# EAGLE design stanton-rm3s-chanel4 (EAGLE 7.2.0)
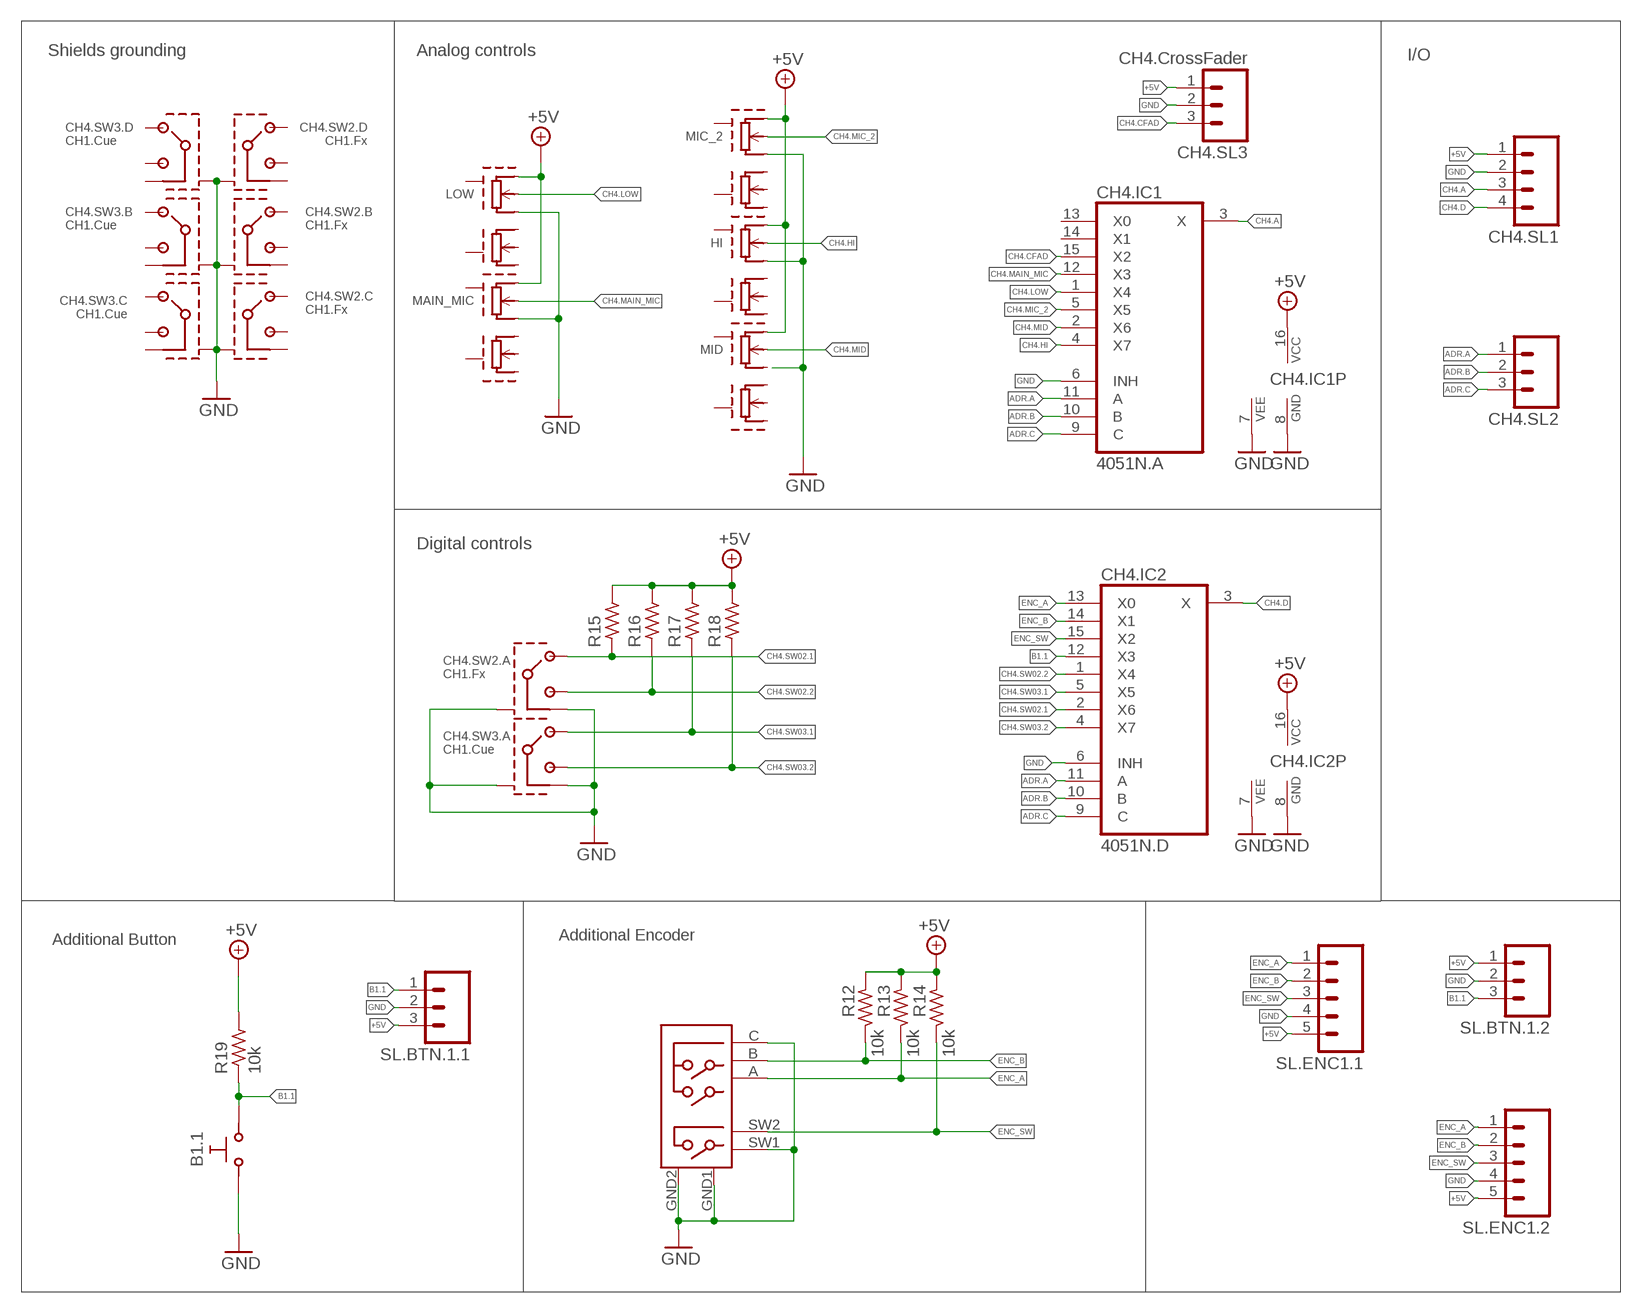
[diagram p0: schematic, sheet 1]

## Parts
B1.1  SW-TAKTSS  [SW_TAKT12X12SS]
CH4.IC1  4051N.A  4051N  [DIL16]
CH4.IC2  4051N.D  4051N  [DIL16]
CH4.SL1  M04  [04P]
CH4.SL2  M03  [03P]
CH4.SL3  CH4.CrossFader  M03  [03P]
CH4.SW2.  CH1.Fx  RM3S-1P-SWITCH  [RM3S-1P-SWITCH]
CH4.SW3.  CH1.Cue  RM3S-1P-SWITCH  [RM3S-1P-SWITCH]
ENC01  STEC  [STEC]
HI  RM3S-POTRM3S-POT  [RM3S-POT]
LOW  RM3S-POTRM3S-POT  [RM3S-POT]
MAIN_MIC  RM3S-POTRM3S-POT  [RM3S-POT]
MIC_2  RM3S-POTRM3S-POT  [RM3S-POT]
MID  RM3S-POTRM3S-POT  [RM3S-POT]
R12  10k  R-EU_0207/10  [0207/10]
R13  10k  R-EU_0207/10  [0207/10]
R14  10k  R-EU_0207/10  [0207/10]
R15  R-EU_0207/10C  [0207/10C]
R16  R-EU_0207/10C  [0207/10C]
R17  R-EU_0207/10C  [0207/10C]
R18  R-EU_0207/10C  [0207/10C]
R19  10k  R-EU_0207/10  [0207/10]
SL.BTN.1.1  M03  [03P]
SL.BTN.1.2  M03  [03P]
SL.ENC1.1  M05  [05P]
SL.ENC1.2  M05  [05P]

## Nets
+5V: CH4.IC1.16(VCC) CH4.IC2.16(VCC) CH4.SL1.1 CH4.SL3.1 HI.1 LOW.1 MAIN_MIC.1 MIC_2.1 MID.1 R12.1 R13.1 R14.1 R15.2 R16.2 R17.2 R18.2 R19.2 SL.BTN.1.1.3 SL.BTN.1.2.1 SL.ENC1.1.5 SL.ENC1.2.5
ADR.A: CH4.IC1.11(A) CH4.IC2.11(A) CH4.SL2.1
ADR.B: CH4.IC1.10(B) CH4.IC2.10(B) CH4.SL2.2
ADR.C: CH4.IC1.9(C) CH4.IC2.9(C) CH4.SL2.3
B1.1: B1.1.P$2 CH4.IC2.12(X3) R19.1 SL.BTN.1.1.1 SL.BTN.1.2.3
CH4.A: CH4.IC1.3(X) CH4.SL1.3
CH4.CFAD: CH4.IC1.15(X2) CH4.SL3.3
CH4.D: CH4.IC2.3(X) CH4.SL1.4
CH4.HI: CH4.IC1.4(X7) HI.6
CH4.LOW: CH4.IC1.1(X4) LOW.6
CH4.MAIN_MIC: CH4.IC1.12(X3) MAIN_MIC.6
CH4.MIC_2: CH4.IC1.5(X5) MIC_2.6
CH4.MID: CH4.IC1.2(X6) MID.6
CH4.SW02.1: CH4.IC2.2(X6) CH4.SW2..1.1 R15.1
CH4.SW02.2: CH4.IC2.1(X4) CH4.SW2..1.3 R16.1
CH4.SW03.1: CH4.IC2.5(X5) CH4.SW3..1.1 R17.1
CH4.SW03.2: CH4.IC2.4(X7) CH4.SW3..1.3 R18.1
ENC_A: CH4.IC2.13(X0) ENC01.A R13.2 SL.ENC1.1.1 SL.ENC1.2.1
ENC_B: CH4.IC2.14(X1) ENC01.B R12.2 SL.ENC1.1.2 SL.ENC1.2.2
ENC_SW: CH4.IC2.15(X2) ENC01.SW2 R14.2 SL.ENC1.1.3 SL.ENC1.2.3
GND: B1.1.P$1 CH4.IC1.6(INH) CH4.IC1.7(VEE) CH4.IC1.8(GND) CH4.IC2.6(INH) CH4.IC2.7(VEE) CH4.IC2.8(GND) CH4.SL1.2 CH4.SL3.2 CH4.SW2..1.4 CH4.SW2..P$13(A:GND1) CH4.SW2..P$14(B:GND1) CH4.SW2..P$15(C:GND1) CH4.SW2..P$16(D:GND1) CH4.SW3..1.4 CH4.SW3..P$13(A:GND1) CH4.SW3..P$14(B:GND1) CH4.SW3..P$15(C:GND1) CH4.SW3..P$16(D:GND1) ENC01.C(COMMON) ENC01.GND1 ENC01.GND2 ENC01.SW1 HI.5 LOW.5 MAIN_MIC.5 MIC_2.5 SL.BTN.1.1.2 SL.BTN.1.2.2 SL.ENC1.1.4 SL.ENC1.2.4
Unconnected: CH4.IC1.13(X0) CH4.IC1.14(X1) CH4.SW2..2.1 CH4.SW2..2.3 CH4.SW2..2.4 CH4.SW2..3.1 CH4.SW2..3.3 CH4.SW2..3.4 CH4.SW2..4.1 CH4.SW2..4.3 CH4.SW2..4.4 CH4.SW3..2.1 CH4.SW3..2.3 CH4.SW3..2.4 CH4.SW3..3.1 CH4.SW3..3.3 CH4.SW3..3.4 CH4.SW3..4.1 CH4.SW3..4.3 CH4.SW3..4.4 HI.2 HI.3 HI.4 HI.GND1 HI.GND2 LOW.2 LOW.3 LOW.4 LOW.GND1 LOW.GND2 MAIN_MIC.2 MAIN_MIC.3 MAIN_MIC.4 MAIN_MIC.GND1 MAIN_MIC.GND2 MIC_2.2 MIC_2.3 MIC_2.4 MIC_2.GND1 MIC_2.GND2 MID.2 MID.3 MID.4 MID.5 MID.GND1 MID.GND2

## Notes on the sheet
- Shields grounding | Analog controls | I/O
- Digital controls
- Additional Button | Additional Encoder

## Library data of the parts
B1.1 = gogo:SW-TAKT
CH4.IC1 CH4.IC2 = 40xx:4051: 8-channel ANALOG MULTIPLEXER
CH4.SL1 = con-amp-quick:M04: AMP QUICK CONNECTOR
CH4.SL2 CH4.SL3 SL.BTN.1.1 SL.BTN.1.2 = con-amp-quick:M03: AMP QUICK CONNECTOR
CH4.SW2. CH4.SW3. = stanton-rm3s:RM3S-1P-SWITCH
ENC01 = rotary-encoder-STUC:STEC
HI LOW MAIN_MIC MIC_2 MID = stanton-rm3s:RM3S-POT
R12-R19 = rcl:R-EU_: RESISTOR, European symbol
SL.ENC1.1 SL.ENC1.2 = con-amp-quick:M05: AMP QUICK CONNECTOR

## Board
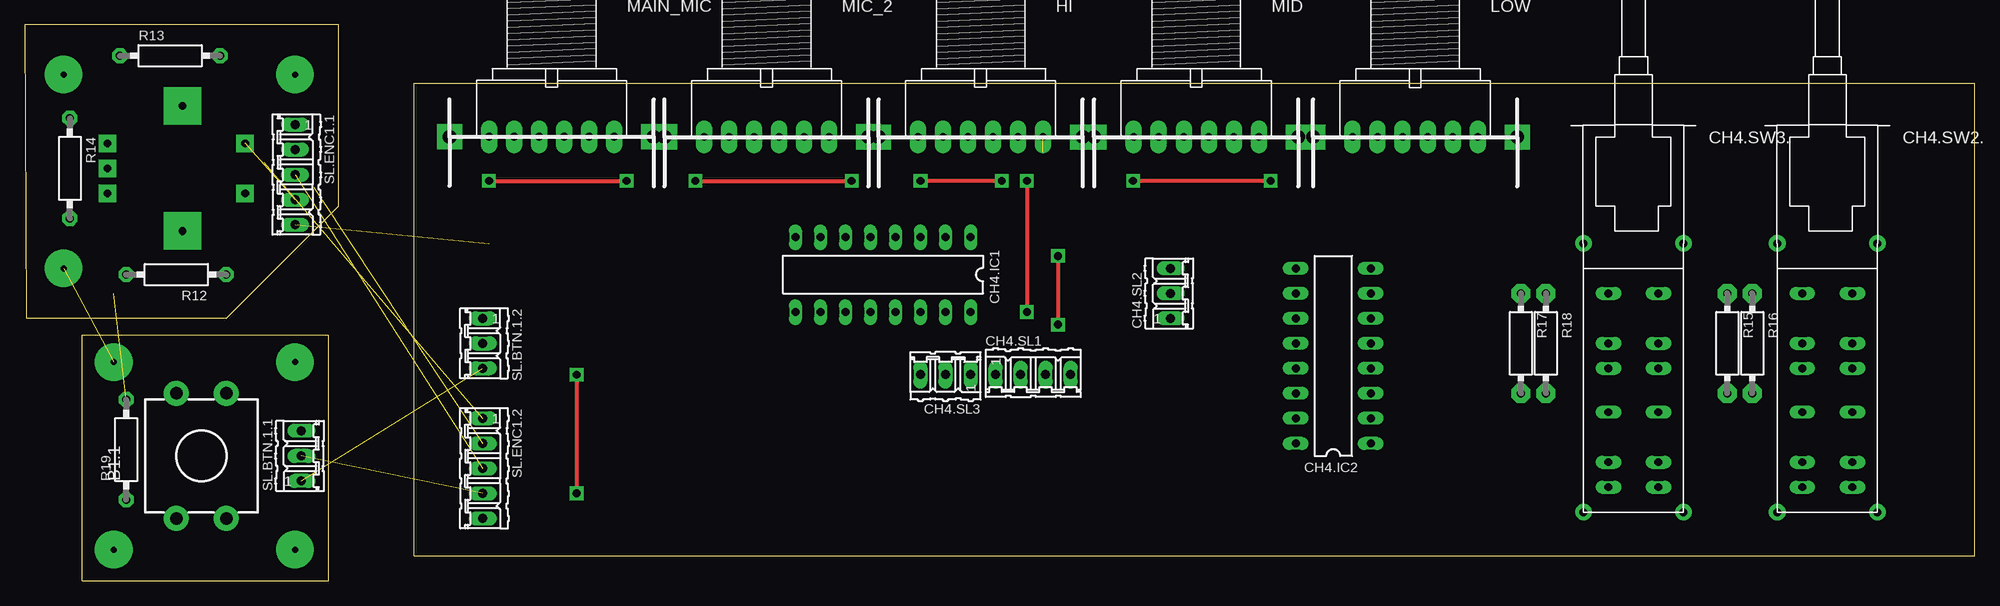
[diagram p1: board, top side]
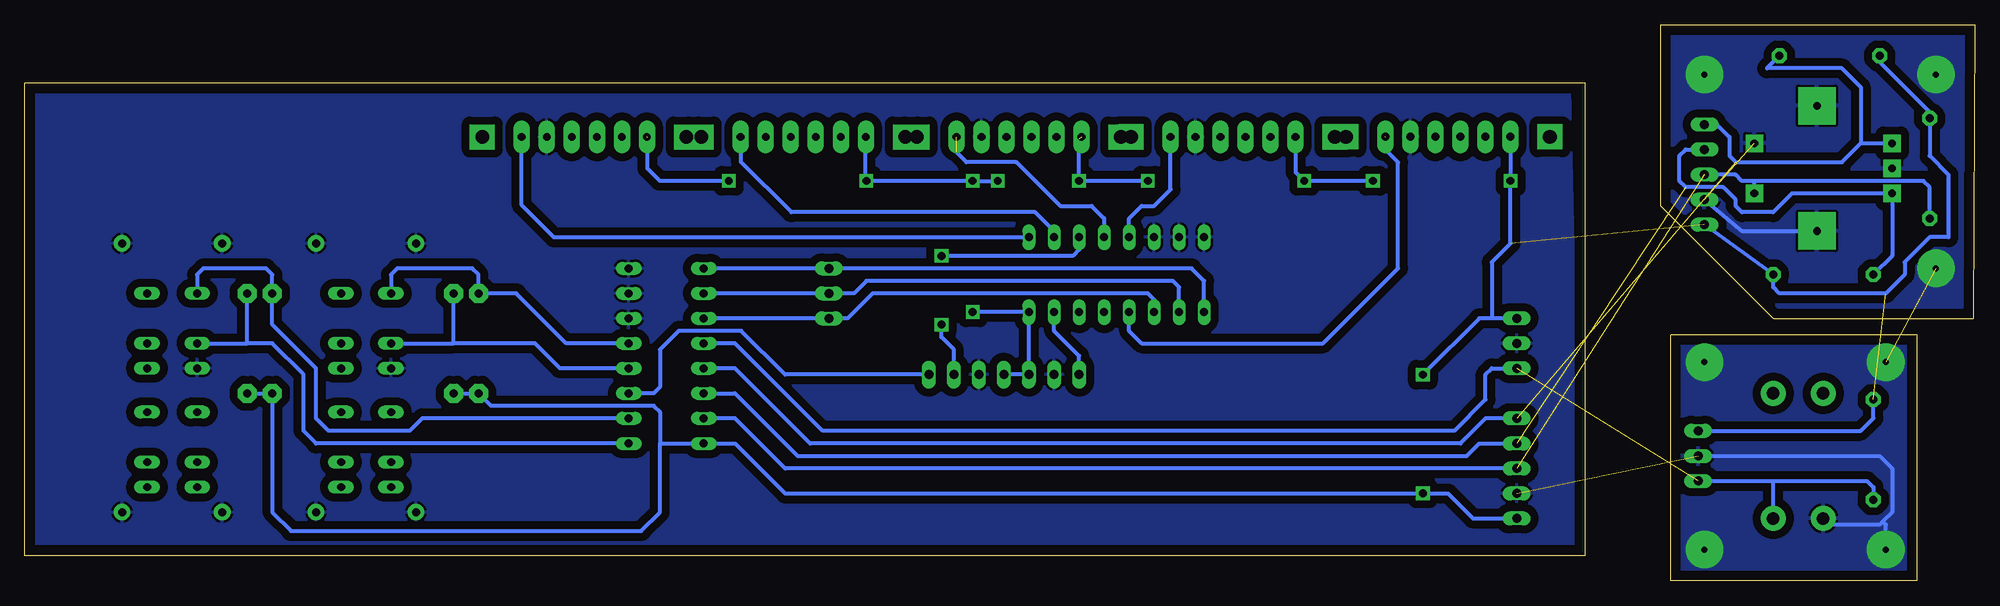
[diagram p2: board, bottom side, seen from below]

Size 198.02 x 56.51 mm. Coordinates in mm from the lower left corner, seen from the top.
Outline: 39.52,2.54 39.52,50.54 198.02,50.54 198.02,2.54 39.52,2.54
Outline: 31.9,56.51 0,56.51 0.15,26.67 20.47,26.67 31.9,38.1 31.9,56.51
Outline: 5.87,0 30.87,0 30.87,25 5.87,25 5.87,0
Copper layers (1*16): Top 0.035mm / dielectric 1.5mm / Bottom 0.035mm
Design rules "default": minimum track width 10mil, minimum drill 24mil, track to track 8mil, track to pad 8mil, pad to pad 8mil, via to via 8mil, smd to smd 8mil, copper to edge 40mil, drill to drill 8mil, minimum pad ring 10mil, minimum via ring 8mil, stop-mask expansion 4mil, vias tented up to drill 0mil, thermal gap 10mil

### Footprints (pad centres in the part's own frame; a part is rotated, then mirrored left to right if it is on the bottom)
SW_TAKT12X12SS = drill 1.27 pad 2.54: P$1 -2.54,-6.35; P$2 2.54,-6.35; P$3 2.54,6.35; P$4 -2.54,6.35
DIL16 = drill 0.813 long: 1 -8.89,-3.81; 2 -6.35,-3.81; 3 -3.81,-3.81; 4 -1.27,-3.81; 5 1.27,-3.81; 6 3.81,-3.81; 7 6.35,-3.81; 8 8.89,-3.81; 9 8.89,3.81; 10 6.35,3.81; 11 3.81,3.81; 12 1.27,3.81; 13 -1.27,3.81; 14 -3.81,3.81; 15 -6.35,3.81; 16 -8.89,3.81
04P = drill 0.914 long: 1 -3.81,0; 2 -1.27,0; 3 1.27,0; 4 3.81,0
03P = drill 0.914 long: 1 -2.54,0; 2 0,0; 3 2.54,0
RM3S-1P-SWITCH = drill 0.8 long: 1.1 -2.54,0; 1.3 -2.54,-5.08; 1.4 -2.54,-7.62; 2.1 2.54,0; 2.3 2.54,-5.08; 2.4 2.54,-7.62; 3.1 -2.54,-12.065; 3.3 -2.54,-17.145; 3.4 -2.54,-19.685; 4.1 2.54,-12.065; 4.3 2.54,-17.145; 4.4 2.54,-19.685 | drill 0.8 pad 1.676: P$13 -5.08,-22.225; P$14 5.08,-22.225; P$15 -5.08,5.08; P$16 5.08,5.08
STEC = drill 0.8 pad 1.778 square: A -2.54,-7.62; B 2.54,-7.62; C 0,-7.62; SW1 -2.54,6.35; SW2 2.54,6.35 | drill 0.8 pad 3.81 square: GND1 -6.35,0; GND2 6.35,0
RM3S-POT = drill 0.8 pad 1.676 long: 1 -6.35,0; 2 -3.81,0; 3 -1.27,0; 4 1.27,0; 5 3.81,0; 6 6.35,0 | drill 1.4 pad 2.54 square: GND1 -10.36,0; GND2 10.36,0
0207/10 = drill 0.813 pad 1.524 octagon: 1 -5.08,0; 2 5.08,0
0207/10C = drill 0.813 pad 1.93 octagon: 1 -5.08,0; 2 5.08,0
05P = drill 0.914 long: 1 -5.08,0; 2 -2.54,0; 3 0,0; 4 2.54,0; 5 5.08,0

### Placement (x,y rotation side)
B1.1  17.94,12.7 0 top
CH4.IC1  87.15,31.11 180 top
CH4.IC2  132.87,22.86 90 top
CH4.SL1  102.39,20.95 0 top
CH4.SL2  116.36,29.21 90 top
CH4.SL3  93.5,20.95 180 top
CH4.SW2.  183.04,29.21 0 top
CH4.SW3.  163.35,29.21 0 top
ENC01  16.03,41.91 270 top
HI  97.06,45.1 0 top
LOW  141.19,45.1 0 top
MAIN_MIC  53.5,45.12 0 top
MIC_2  75.32,45.11 0 top
MID  118.96,45.11 0 top
R12  15.39,31.11 180 top
R13  14.76,53.34 0 top
R14  4.6,41.91 270 top
R15  172.87,24.13 270 top
R16  175.42,24.13 270 top
R17  151.92,24.13 270 top
R18  154.46,24.13 270 top
R19  10.31,13.33 90 top
SL.BTN.1.1  28.09,12.7 90 top
SL.BTN.1.2  46.51,24.13 270 top
SL.ENC1.1  27.46,41.27 270 top
SL.ENC1.2  46.51,11.43 270 top

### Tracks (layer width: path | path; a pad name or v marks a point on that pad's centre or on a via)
+5V  (via drill 0.8 pad 1.4)  (4 unrouted)
  Top 0.406: v99.21,40.64 v90.96,40.64 | v101.75,40.64 v101.75,27.3 | v47.14,40.64 v61.12,40.64 | v68.1,40.64 v83.97,40.64 | v126.52,40.64 v112.55,40.64 | v56.03,20.95 v56.03,8.89
  Bottom 0.406: R18.2 R17.2 150.65,17.78 134.14,17.78 133.5,17.14 133.5,13.97 | 133.5,13.97 133.5,6.98 135.41,5.08 170.97,5.08 172.87,6.98 R15.2 R16.2 | v99.21,40.64 v101.75,40.64 v112.55,40.64 112.63,40.72 112.63,45.08 MID.1 | 90.96,44.86 v90.96,40.64 v83.97,40.64 | v61.12,40.64 v68.1,40.64 68.97,41.51 MIC_2.1 | 133.5,13.97 CH4.IC2.16 125.88,13.97 120.81,8.89 v56.03,8.89 53.5,8.89 50.95,6.35 SL.ENC1.2.5 | SL.BTN.1.2.1 49.05,26.67 | 49.05,26.67 49.05,32.38 47.14,34.29 v47.14,40.64 v47.15,40.65 MAIN_MIC.1 | v126.52,40.64 133.5,40.64 134.77,41.91 134.77,45.03 | SL.ENC1.1.5 R12.1 20.47,29.84 19.84,29.21 9.05,29.21 7.14,31.11 7.14,32.38 4.6,34.92 2.69,34.92 2.69,41.27 4.6,43.18 R14.1 4.6,47.62 9.68,52.7 R13.1 | SL.BTN.1.1.3 11.58,15.24 10.31,16.51 R19.2 | CH4.SL1.1 CH4.SL3.1 CH4.IC1.16 v101.75,27.3 | 49.05,26.67 50.32,26.67 v56.03,20.95
ADR.A
  Bottom 0.406: CH4.IC1.11 83.34,28.57 83.97,29.21 111.92,29.21 114.45,26.67 CH4.SL2.1 CH4.IC2.11
ADR.B
  Bottom 0.406: CH4.IC1.10 80.8,29.84 81.44,30.48 112.55,30.48 113.82,29.21 CH4.SL2.2 CH4.IC2.10
ADR.C
  Bottom 0.406: CH4.IC1.9 78.26,30.48 79.53,31.75 CH4.SL2.3 CH4.IC2.9
B1.1  (1 unrouted)
  Bottom 0.406: CH4.IC2.12 125.88,24.13 117,15.24 52.86,15.24 49.69,18.41 49.69,20.95 49.05,21.59 SL.BTN.1.2.3 | SL.BTN.1.1.1 20.47,10.16 | 20.47,10.16 10.95,10.16 10.31,9.52 R19.1 | B1.1.P$2 20.47,10.16
CH4.A  (via drill 0.8 pad 1.4)
  Top 0.406: v104.93,33.02 v104.93,26.03
  Bottom 0.406: CH4.IC1.3 90.96,33.66 91.59,33.02 v104.93,33.02 | CH4.SL1.3 103.66,23.49 104.93,24.76 v104.93,26.03
CH4.CFAD
  Bottom 0.406: CH4.SL3.3 90.96,22.86 93.5,25.4 CH4.IC1.15
CH4.D
  Bottom 0.406: CH4.SL1.4 120.81,20.95 125.25,25.4 131.6,25.4 133.5,23.49 133.5,19.69 134.14,19.05 CH4.IC2.3
CH4.HI  (1 unrouted)
  Bottom 0.406: CH4.IC1.4 88.42,36.83 89.69,38.1 92.87,38.1 97.31,42.54 102.39,42.54 103.42,43.57
CH4.LOW
  Bottom 0.406: CH4.IC1.1 144.3,34.92 147.53,38.16 LOW.6
CH4.MAIN_MIC  (1 unrouted)
  Bottom 0.406: CH4.IC1.12 85.88,25.4 84.61,24.13 66.19,24.13 58.57,31.75 58.57,42.54 59.84,43.81 59.84,45.11
CH4.MIC_2
  Bottom 0.406: CH4.IC1.5 85.88,36.83 84.61,38.1 83.34,38.1 81.67,39.77 MIC_2.6
CH4.MID
  Bottom 0.406: CH4.IC1.2 93.5,35.56 95.4,37.47 120.17,37.47 125.31,42.6 MID.6
CH4.SW02.1
  Bottom 0.406: CH4.IC2.2 157.63,16.51 158.9,15.24 167.16,15.24 168.43,16.51 168.43,21.59 172.87,26.03 R15.1 172.87,31.11 173.51,31.75 179.86,31.75 180.49,31.11 CH4.SW2..1.1
CH4.SW02.2
  Bottom 0.406: CH4.SW2..1.3 175.42,24.13 | 175.42,24.13 R16.1 | CH4.IC2.1 168.43,13.97 169.7,15.24 169.7,20.95 172.87,24.13 175.42,24.13
CH4.SW03.1
  Bottom 0.406: CH4.IC2.5 143.03,24.13 148.11,29.21 R17.1 151.92,31.11 152.56,31.75 160.18,31.75 160.81,31.11 CH4.SW3..1.1
CH4.SW03.2
  Bottom 0.406: CH4.SW3..1.3 154.46,24.13 | 154.46,24.13 146.2,24.13 143.67,21.59 CH4.IC2.4 | 154.46,24.13 R18.1
ENC_A  (1 unrouted)
  Bottom 0.406: SL.ENC1.2.1 49.69,16.51 52.22,13.97 118.26,13.97 125.88,21.59 CH4.IC2.13 | 8.41,45.08 ENC01.A 11.58,44.45 | R13.2 21.11,52.07 13.49,52.07 11.58,50.16 11.58,44.45 | SL.ENC1.1.1 26.19,46.35 24.92,45.08 24.92,43.18 24.28,42.54 13.49,42.54 11.58,44.45
ENC_B  (1 unrouted)
  Bottom 0.406: CH4.IC2.14 125.88,19.05 119.53,12.7 51.59,12.7 50.32,13.97 SL.ENC1.2.2 | R12.2 8.41,33.02 ENC01.B 18.57,39.37 20.47,37.47 23.65,37.47 24.28,38.1 24.28,38.73 25.56,40 29.37,40 30,40.64 30,43.18 29.37,43.81 SL.ENC1.1.2
ENC_SW  (1 unrouted)
  Bottom 0.406: CH4.IC2.15 125.88,16.51 120.81,11.43 SL.ENC1.2.3 | R14.2 4.6,40 5.24,40.64 22.38,40.64 | 22.38,40.64 23.65,40.64 24.28,41.27 SL.ENC1.1.3 | ENC01.SW2 22.38,40.64
GND  (via drill 0.6 pad 3.81)  (3 unrouted)
  Bottom 0.406: SL.ENC1.1.4 23.65,35.56 ENC01.GND2 | SL.BTN.1.1.2 9.68,12.7 8.41,11.43 8.41,6.98 9.36,6.03 | 9.36,6.03 9.68,5.72 14.76,5.72 B1.1.P$1 | v9.05,3.17 9.05,5.72 9.36,6.03
  other vias: 3.96,31.75 9.05,22.22 27.46,22.22 27.46,3.17 3.96,51.44 27.46,51.44
  pour Bottom (isolate 0.813): 41.16,50.07 40.16,3.17 197,3.17 198,50.07
  pour Bottom (isolate 0.813): 0.15,56.51 0.15,26.67 20.47,26.67 31.9,38.1 31.9,56.51
  pour Bottom (isolate 0.813): 5.87,24.76 30.63,24.76 30.63,0 5.87,0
